PROGRAM p09_casovniki
VAR
	casovnikTP: TP;
	casovnikTON: TON;
	casovnikTOF: TOF;
	vrednostTP: TIME;
	vrednostTON: TIME;
	vrednostTOF: TIME;
	S0: BOOL;	
	L0: BOOL;
	L1: BOOL;
	L2: BOOL;
END_VAR

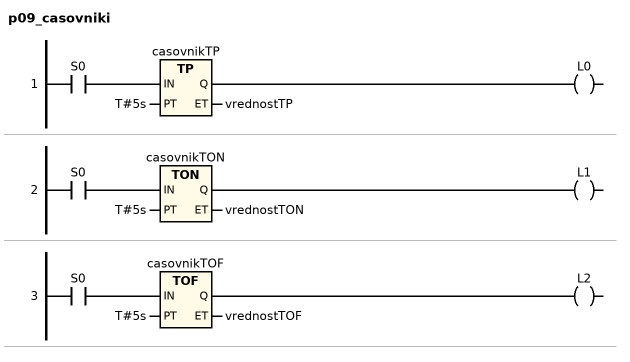
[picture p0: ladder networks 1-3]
// NETWORK 1
casovnikTP(IN := S0, PT := T#5s, ET => vrednostTP); // TP
L0 := casovnikTP.Q;

// NETWORK 2
casovnikTON(IN := S0, PT := T#5s, ET => vrednostTON); // TON
L1 := casovnikTON.Q;

// NETWORK 3
casovnikTOF(IN := S0, PT := T#5s, ET => vrednostTOF); // TOF
L2 := casovnikTOF.Q;

END_PROGRAM
